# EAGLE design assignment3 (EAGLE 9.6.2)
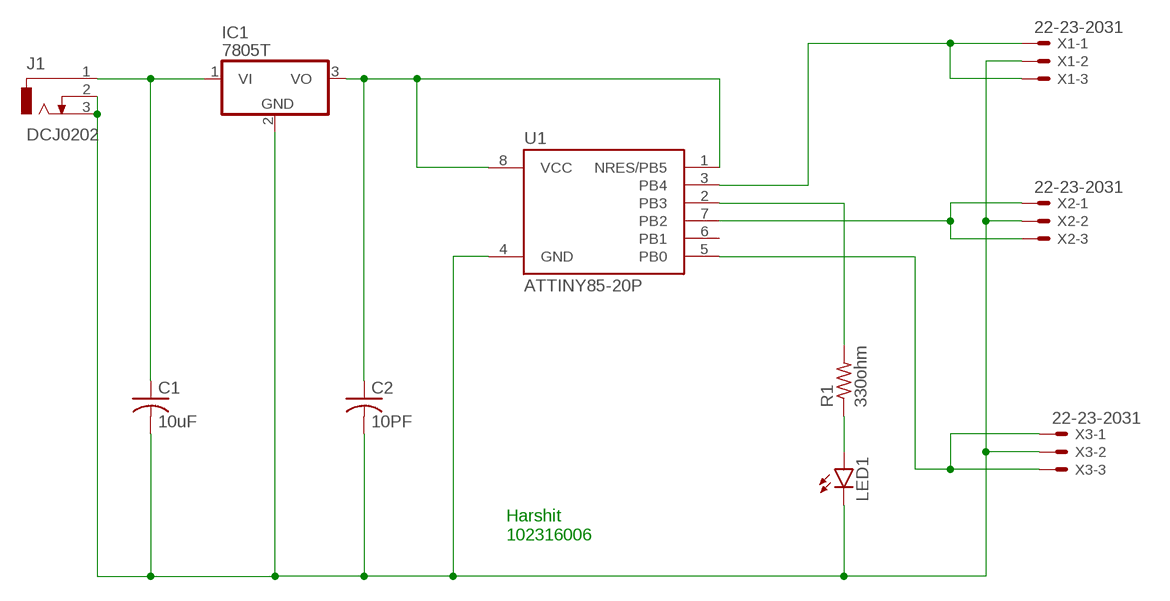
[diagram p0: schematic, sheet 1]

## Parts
C1  10uF  C-US025-024X044  [C025-024X044]
C2  10PF  C-US025-024X044  [C025-024X044]
IC1  7805T  [TO220H]
J1  DCJ0202  [DCJ0202]
LED1  LED3MM  [LED3MM]
R1  330ohm  R-US_0207/5V  [0207/5V]
U1  ATTINY85-20P  [PDIP08_300MIL]
X1  22-23-2031  [22-23-2031]
X2  22-23-2031  [22-23-2031]
X3  22-23-2031  [22-23-2031]

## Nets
N$1: C1.1 IC1.1(VI) J1.1
N$2: C1.2 C2.2 IC1.2(GND) J1.2 J1.3 LED1.K(C) U1.4(GND) X1.2 X2.2 X3.2
N$3: C2.1 IC1.3(VO) U1.1(NRES/PB5) U1.8(VCC)
N$4: U1.3(PB4) X1.1 X1.3
N$5: U1.5(PB0) X3.1 X3.3
N$7: R1.2 U1.2(PB3)
N$8: LED1.A R1.1
N$10: U1.7(PB2) X2.1 X2.3
Unconnected: U1.6(PB1)

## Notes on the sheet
- Harshit
  102316006

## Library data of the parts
C1 C2 = rcl:C-US: CAPACITOR, American symbol; SPICEPREFIX: C
IC1 = linear:78*: Positive VOLTAGE REGULATOR Source: http://cache.national.com/ds/LM/LM78L05.pdf http://www.fairchildsemi.com/ds/LM/LM7805.pdf
J1 = con-jack:DCJ0202: DC POWER JACK Source: DCJ0202.pdf; OC_FARNELL: unknown; OC_NEWARK: unknown
LED1 = led:LED: LED
R1 = rcl:R-US_: RESISTOR, American symbol; SPICEPREFIX: R
U1 = _hhn_attiny25_45_85:ATTINY85*: ATMEL ATtiny 85 Packages: P = PDIP 08 30mil S = SOIC 08 EIAJ 208mil Technologies Note: for complete ordering code (temp. range, finish, tape&reel etc.) see www.atmel.com &bull; Supply Voltage: V = (1.8&hellip;5.5)V | [blank] = (2.7&hellip;5.5)V &bull; Speed: 10 = 10 MHz | 20 = 20 MHz Author: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
X1-X3 = con-molex:22-23-2031: .100" (2.54mm) Center Header - 3 Pin; MF: MOLEX; MPN: 22-23-2031; OC_FARNELL: 1462950; OC_NEWARK: 30C0862

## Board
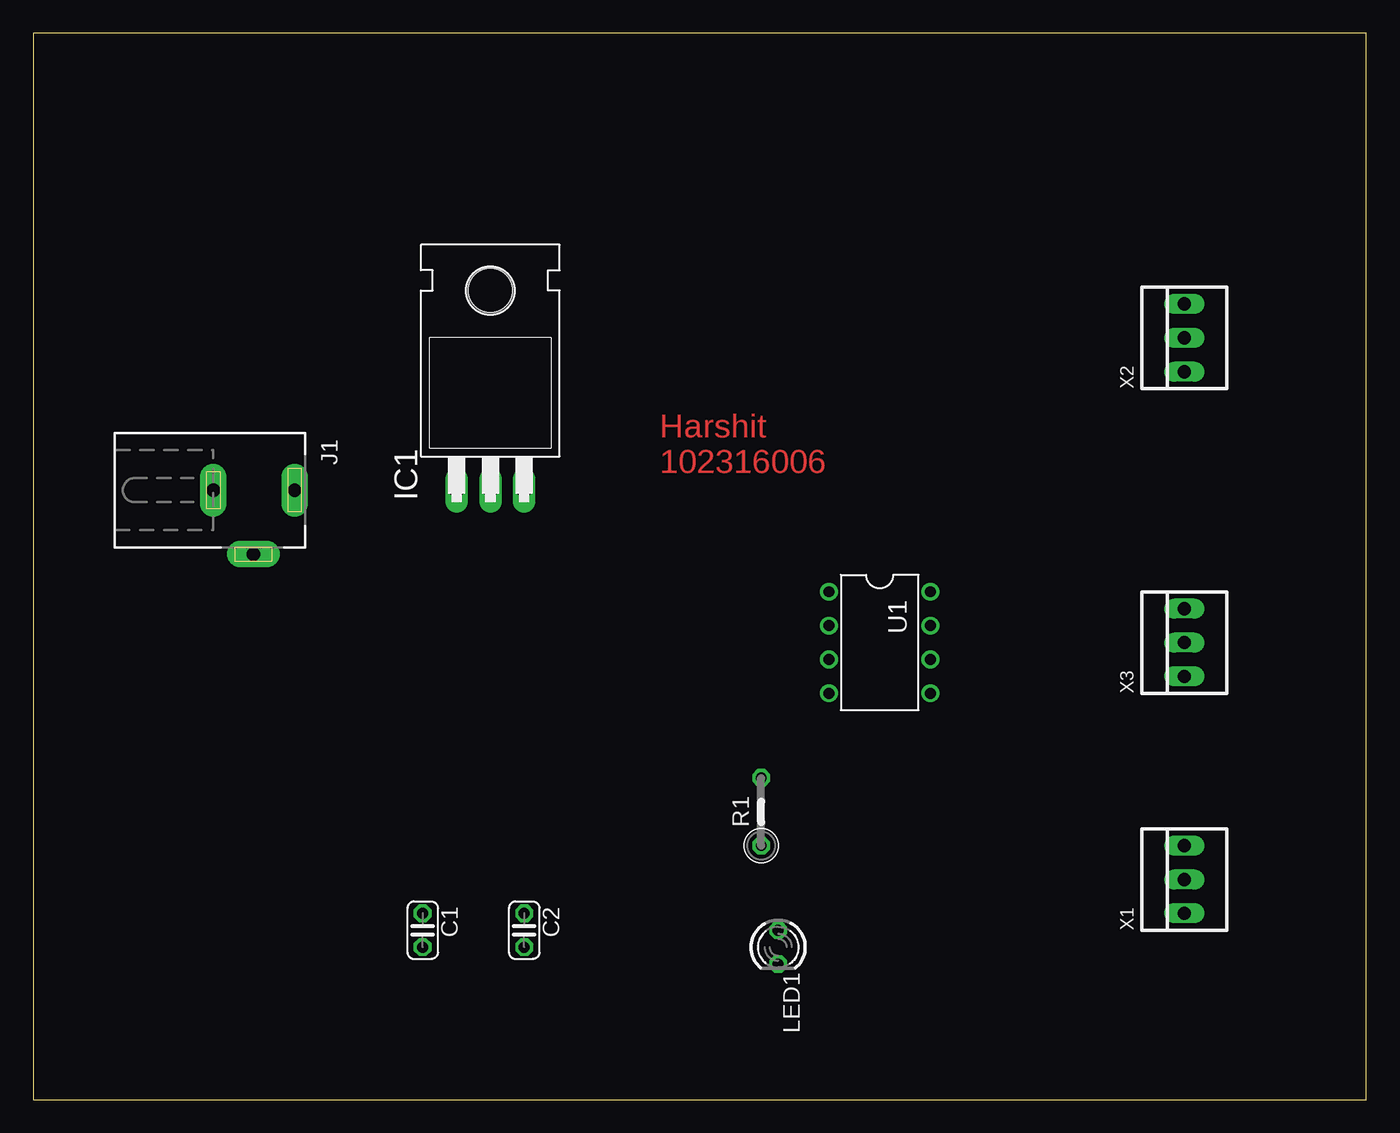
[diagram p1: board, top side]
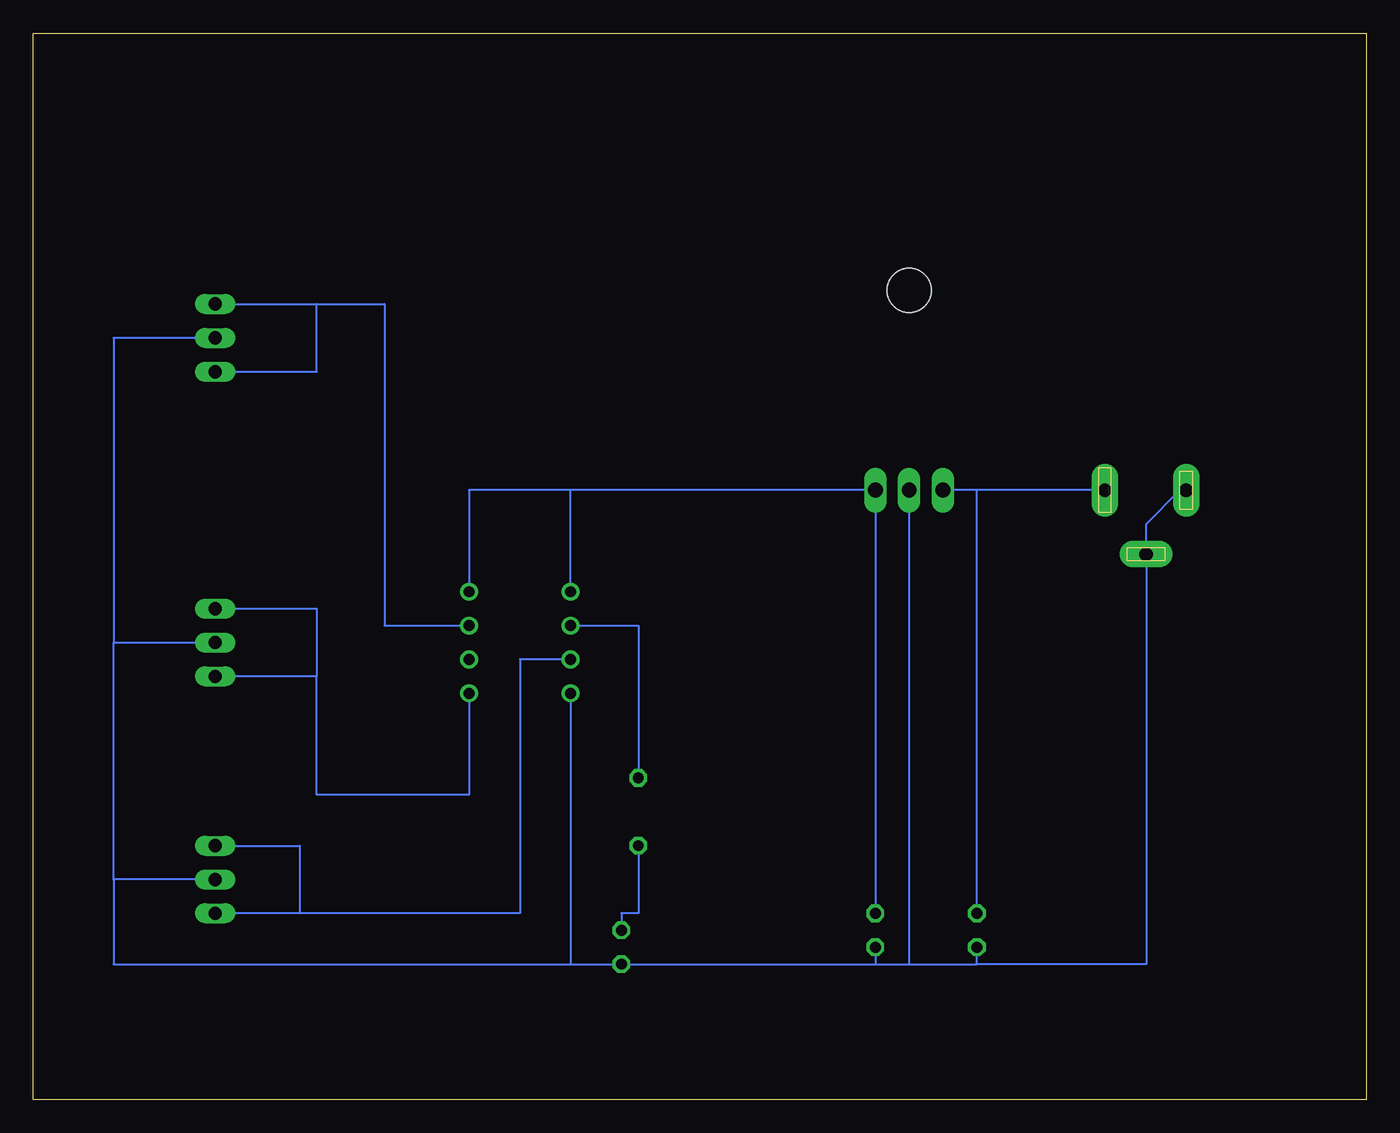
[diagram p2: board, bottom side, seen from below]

Size 100 x 80 mm. Coordinates in mm from the lower left corner, seen from the top.
Outline: 0,0 100,0 100,80 0,80 0,0
Copper layers (1*16): Top 0.035mm / dielectric 1.5mm / Bottom 0.035mm
Design rules "default": minimum track width 6mil, minimum drill 0.35mm, track to track 6mil, track to pad 6mil, pad to pad 6mil, via to via 6mil, smd to smd 6mil, copper to edge 40mil, drill to drill 6mil, minimum pad ring 10mil, minimum via ring 8mil, stop-mask expansion 4mil, vias tented up to drill 0mil, thermal gap 10mil

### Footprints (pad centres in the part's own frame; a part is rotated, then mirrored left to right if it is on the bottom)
C025-024X044 = drill 0.813 octagon: 1 -1.27,0; 2 1.27,0
TO220H = drill 1.118 long: 1 -2.54,-10.16; 2 0,-10.16; 3 2.54,-10.16 | hole 3.302: 0,4.826
DCJ0202 = drill 1 pad 2 long: 1 0,3.1; 2 4.8,0; 3 0,-3
LED3MM = drill 0.813 octagon: A -1.27,0; K 1.27,0
0207/5V = drill 0.813 octagon: 1 -2.54,0; 2 2.54,0
PDIP08_300MIL = drill 0.813: 1 -3.81,-3.81; 2 -1.27,-3.81; 3 1.27,-3.81; 4 3.81,-3.81; 5 3.81,3.81; 6 1.27,3.81; 7 -1.27,3.81; 8 -3.81,3.81
22-23-2031 = drill 1 long: 1 -2.54,0; 2 0,0; 3 2.54,0

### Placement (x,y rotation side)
C1  29.21,12.7 270 top
C2  36.83,12.7 270 top
IC1  34.29,55.88 0 top
J1  16.51,45.72 270 top
LED1  55.88,11.43 270 top
R1  54.61,21.59 90 top
U1  63.5,34.29 270 top
X1  86.36,16.51 90 top
X2  86.36,57.15 90 top
X3  86.36,34.29 90 top

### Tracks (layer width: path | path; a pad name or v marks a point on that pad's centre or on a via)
N$1
  Bottom 0.152: J1.1 29.21,45.72 | 29.21,45.72 IC1.1 | C1.1 29.21,45.72
N$2
  Bottom 0.152: 36.83,10.16 LED1.K 59.69,10.16 | C2.2 36.83,10.16 | 36.83,10.16 34.29,10.16 | 34.29,10.16 29.21,10.16 | 29.21,10.16 C1.2 | J1.3 13.97,45.72 16.51,43.18 J1.2 16.51,10.16 29.21,10.16 | IC1.2 34.29,10.16 | X2.2 93.98,57.15 93.98,34.29 | 93.98,34.29 X3.2 | X1.2 93.98,16.51 | 93.98,16.51 93.98,34.29 | U1.4 59.69,10.16 | 93.98,16.51 93.98,10.16 59.69,10.16
N$3
  Bottom 0.152: C2.1 IC1.3 59.69,45.72 | 59.69,45.72 67.31,45.72 U1.8 | U1.1 59.69,45.72
N$4
  Bottom 0.152: U1.3 63.5,33.02 63.5,13.97 80.01,13.97 | 80.01,13.97 X1.1 | X1.3 80.01,19.05 80.01,13.97
N$5
  Bottom 0.152: X3.3 78.74,36.83 78.74,31.75 | 78.74,31.75 X3.1 | U1.5 67.31,22.86 78.74,22.86 78.74,31.75
N$7
  Bottom 0.152: U1.2 54.61,35.56 R1.2
N$8
  Bottom 0.152: R1.1 54.61,13.97 55.88,13.97 LED1.A
N$10
  Bottom 0.152: X2.3 78.74,59.69 | 78.74,59.69 73.66,59.69 73.66,35.56 U1.7 | X2.1 78.74,54.61 78.74,59.69

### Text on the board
Top: Harshit / 102316006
